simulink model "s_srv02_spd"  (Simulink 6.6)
settings: Solver=ode4  SolverMode=SingleTasking  StartTime=0.0  StopTime=5  FixedStep=0.0002  RelTol=1e-3  AbsTol=1e-6
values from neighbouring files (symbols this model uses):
  a = 10^(-21/20)    (= 0.0891250938134)    [d_lag_q3.m]    (also in d_lead.m = (1+sin(phi_m)) / (1-sin(phi_m)); setup_srv02_exp03_spd.m = 1)
  bsp = 0    [setup_srv02_exp03_spd.m]
  K = Am / Beq_v    [d_model_param.m]    (also in setup_srv02_exp01_mdl.m = 1)
  K_AMP = 1    [setup_srv02_exp03_spd.m]    (also in setup_srv02_exp01_mdl.m; setup_srv02_exp02_pos.m)
  Kc = 10^(e_ss_meas/e_ss_min/20)    (= 2.14783047413)    [d_lag_q3.m]    (also in d_lead.m = 53.0884444231; setup_srv02_exp03_spd.m = 0)
  ki = wn^2*tau/K    [d_pi_design.m]    (also in setup_srv02_exp03_spd.m = 0; d_i_design.m = -( -AmpMax + kp * e_ss ) / ti / e_ss; setup_srv02_exp02_pos.m = 0)
  kp = (-1+2*zeta*wn*tau)/K    [d_pi_design.m]    (also in setup_srv02_exp03_spd.m = 0; d_pv_design.m = wn^2/K*tau; setup_srv02_exp02_pos.m = 0)
  T = 10 / (wg_des * a)    [d_lag_q3.m]    (also in d_lead.m = 1 / (w_m * sqrt(a)); setup_srv02_exp03_spd.m = 1)
  tau = Jeq / Beq_v    [d_model_param.m]    (also in setup_srv02_exp01_mdl.m = 0.1)
  VMAX_AMP = 0    [config_srv02.m]
  VMAX_DAC = 10    [setup_srv02_exp03_spd.m]    (also in setup_srv02_exp01_mdl.m; setup_srv02_exp02_pos.m)
undefined symbols (not defined in the file or in its folder): square
libraries: simulink x3

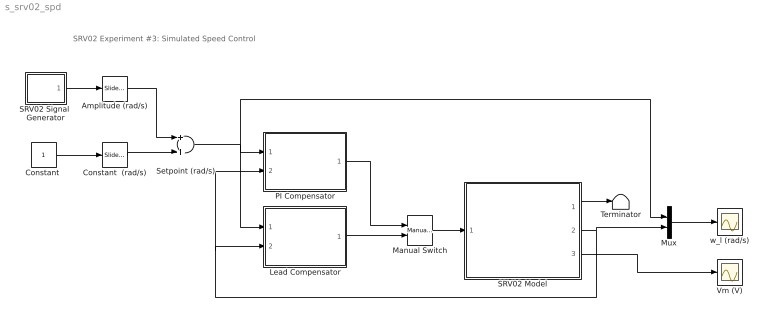
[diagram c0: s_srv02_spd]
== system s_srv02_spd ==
  note: SRV02 Experiment #3: Simulated Speed Control
  Amplitude (rad/s) : simulink/Math Operations/Slider Gain  SystemSampleTime=-1  low=0  gain=5  high=10
  "Constant " : Constant
  Constant  (rad/s) : simulink/Math Operations/Slider Gain  SystemSampleTime=-1  low=0  gain=10  high=20
  Lead Compensator : Subsystem
  Manual Switch : simulink/Signal Routing/Manual Switch  SystemSampleTime=-1  sw=1  action=0  varsize=off
  Mux : Mux  Inputs=2
  PI Compensator : Subsystem
  SRV02 Model : Subsystem
  SRV02 Signal  Generator : Subsystem  mask(QET Signal Generator){sig_type=square, a=1, f=0.4}
      mask prompts: sig_type "Signal Type"; a "Amplitude"; f "Frequency (Hz)"
      mask help: Generates a square, triangular, or sinusoidal waveform of a specified amplitude and frequency.
  Setpoint (rad/s) : Sum  OutScaling=2^-10
  Terminator : Terminator
  Vm (V) : Scope
  w_l (rad/s) : Scope
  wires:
  Setpoint (rad/s)/1 -> Mux/1, PI Compensator/1(wd (rad/s)), Lead Compensator/1(wd (rad/s))
  Manual Switch/1 -> SRV02 Model/1(Vi (V))
  SRV02 Model/2(omega_l (rad/s)) -> Mux/2, PI Compensator/2(wl (rad)), Lead Compensator/2(wl (rad/s))
  Mux/1 -> w_l (rad/s)/1
  SRV02 Model/3(Vm (V)) -> Vm (V)/1
  SRV02 Model/1(theta_l (rad)) -> Terminator/1
  Lead Compensator/1(Vi (V)) -> Manual Switch/2
  PI Compensator/1(Vi (V)) -> Manual Switch/1
  SRV02 Signal  Generator/1(out) -> Amplitude (rad/s)/1
  Amplitude (rad/s)/1 -> Setpoint (rad/s)/1
  "Constant "/1 -> Constant  (rad/s)/1
  Constant  (rad/s)/1 -> Setpoint (rad/s)/2

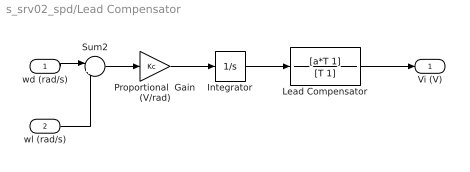
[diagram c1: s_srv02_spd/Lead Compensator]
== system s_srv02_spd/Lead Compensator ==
  wd (rad/s) : Inport
  wl (rad/s) : Inport  Port=2
  Integrator : Integrator
  Lead Compensator : TransferFcn  Numerator=[a*T 1]  Denominator=[T 1]
  Proportional  Gain (V/rad) : Gain  Gain=Kc
  Sum2 : Sum  Inputs=|+-
  Vi (V) : Outport
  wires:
  Lead Compensator/1 -> Vi (V)/1
  Proportional  Gain (V/rad)/1 -> Integrator/1
  Integrator/1 -> Lead Compensator/1
  Sum2/1 -> Proportional  Gain (V/rad)/1
  wd (rad/s)/1 -> Sum2/1
  wl (rad/s)/1 -> Sum2/2

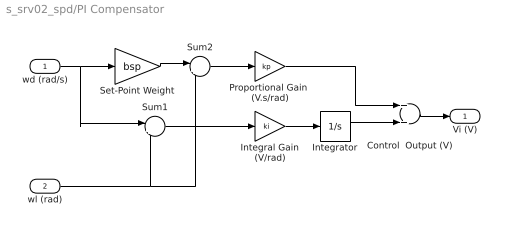
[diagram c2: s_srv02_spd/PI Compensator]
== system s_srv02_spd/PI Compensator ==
  wd (rad/s) : Inport
  wl (rad) : Inport  Port=2
  Control  Output (V) : Sum  OutScaling=2^-10
  Integral Gain (V/rad) : Gain  Gain=ki
  Integrator : Integrator  UpperSaturationLimit=10  LowerSaturationLimit=-10
  Proportional Gain  (V.s/rad) : Gain  Gain=kp
  Set-Point Weight : Gain  Gain=bsp
  Sum1 : Sum  Inputs=|+-
  Sum2 : Sum  Inputs=|+-
  Vi (V) : Outport
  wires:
  Sum1/1 -> Integral Gain (V/rad)/1
  Integral Gain (V/rad)/1 -> Integrator/1
  Integrator/1 -> Control  Output (V)/2
  Proportional Gain  (V.s/rad)/1 -> Control  Output (V)/1
  Set-Point Weight/1 -> Sum2/1
  Sum2/1 -> Proportional Gain  (V.s/rad)/1
  wd (rad/s)/1 -> Set-Point Weight/1, Sum1/1
  Control  Output (V)/1 -> Vi (V)/1
  wl (rad)/1 -> Sum1/2, Sum2/2

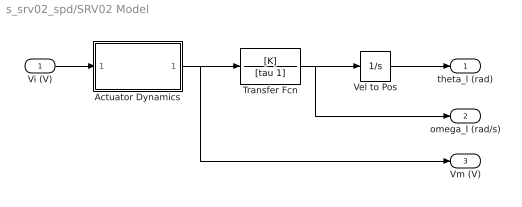
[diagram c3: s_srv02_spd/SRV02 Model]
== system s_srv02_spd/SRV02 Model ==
  Vi (V) : Inport
  Actuator Dynamics : Subsystem
  Transfer Fcn : TransferFcn  Numerator=[K]  Denominator=[tau 1]
  Vel to Pos : Integrator
  theta_l (rad) : Outport
  omega_l (rad/s) : Outport  Port=2
  Vm (V) : Outport  Port=3
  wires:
  Vel to Pos/1 -> theta_l (rad)/1
  Transfer Fcn/1 -> Vel to Pos/1, omega_l (rad/s)/1
  Actuator Dynamics/1(Vm (V)) -> Transfer Fcn/1, Vm (V)/1
  Vi (V)/1 -> Actuator Dynamics/1(Vi (V))

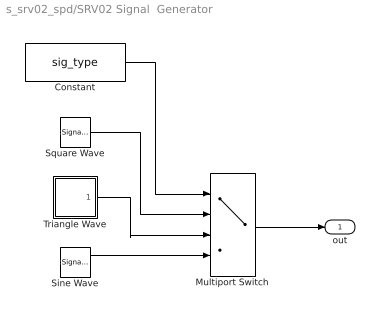
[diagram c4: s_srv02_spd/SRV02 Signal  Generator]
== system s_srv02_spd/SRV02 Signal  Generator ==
  Constant : Constant  Value=sig_type
  Multiport Switch : MultiPortSwitch  Inputs=3
  Sine Wave : SignalGenerator  Amplitude=a  Frequency=f
  Square Wave : SignalGenerator  WaveForm=square  Amplitude=a  Frequency=f
  Triangle Wave : Subsystem
  out : Outport
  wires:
  Square Wave/1 -> Multiport Switch/2
  Triangle Wave/1(out) -> Multiport Switch/3
  Sine Wave/1 -> Multiport Switch/4
  Multiport Switch/1 -> out/1
  Constant/1 -> Multiport Switch/1

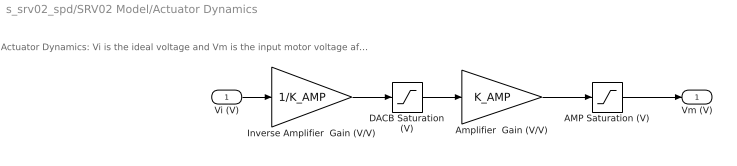
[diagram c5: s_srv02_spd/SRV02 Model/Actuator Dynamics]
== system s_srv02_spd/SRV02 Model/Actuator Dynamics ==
  note: Actuator Dynamics: Vi is the ideal voltage and Vm is the input motor voltage after going through the DACB and amplifier limitiations.
  Vi (V) : Inport
  AMP Saturation (V) : Saturate  UpperLimit=VMAX_AMP  LowerLimit=-VMAX_AMP
  Amplifier  Gain (V/V) : Gain  Gain=K_AMP
  DACB Saturation (V) : Saturate  UpperLimit=VMAX_DAC  LowerLimit=-VMAX_DAC
  Inverse Amplifier  Gain (V/V) : Gain  Gain=1/K_AMP
  Vm (V) : Outport
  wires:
  Inverse Amplifier  Gain (V/V)/1 -> DACB Saturation (V)/1
  DACB Saturation (V)/1 -> Amplifier  Gain (V/V)/1
  Amplifier  Gain (V/V)/1 -> AMP Saturation (V)/1
  Vi (V)/1 -> Inverse Amplifier  Gain (V/V)/1
  AMP Saturation (V)/1 -> Vm (V)/1

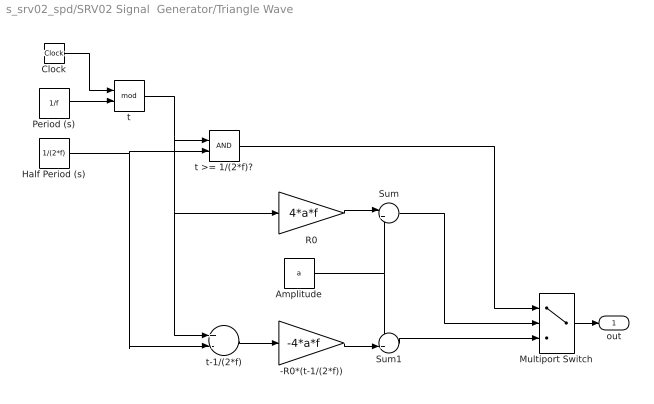
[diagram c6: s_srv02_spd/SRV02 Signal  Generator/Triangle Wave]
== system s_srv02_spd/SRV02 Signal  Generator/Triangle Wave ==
  -R0*(t-1/(2*f)) : Gain  Gain=-4*a*f
  Amplitude : Constant  Value=a
  Clock : Clock
  Half Period (s) : Constant  Value=1/(2*f)
  Multiport Switch : MultiPortSwitch  Inputs=2  zeroidx=on
  Period (s) : Constant  Value=1/f
  R0 : Gain  Gain=4*a*f
  Sum : Sum  Inputs=|+-
  Sum1 : Sum  Inputs=++|
  t : Math  Operator=mod
  t >= 1/(2*f)? : RelationalOperator  LogicOutDataTypeMode=Boolean
  t-1/(2*f) : Sum  Inputs=+-  OutScaling=2^-10
  out : Outport
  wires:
  Sum1/1 -> Multiport Switch/3
  Sum/1 -> Multiport Switch/2
  t >= 1/(2*f)?/1 -> Multiport Switch/1
  -R0*(t-1/(2*f))/1 -> Sum1/2
  Amplitude/1 -> Sum1/1, Sum/2
  R0/1 -> Sum/1
  t-1/(2*f)/1 -> -R0*(t-1/(2*f))/1
  Half Period (s)/1 -> t-1/(2*f)/2, t >= 1/(2*f)?/2
  t/1 -> t-1/(2*f)/1, R0/1, t >= 1/(2*f)?/1
  Period (s)/1 -> t/2
  Clock/1 -> t/1
  Multiport Switch/1 -> out/1
